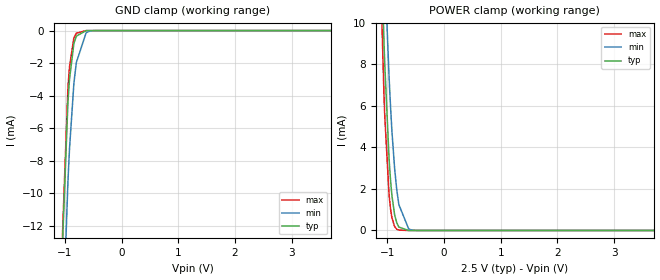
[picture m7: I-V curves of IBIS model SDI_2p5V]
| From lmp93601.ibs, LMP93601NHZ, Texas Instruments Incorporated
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|   Model SDI_2p5V
[Model]   SDI_2p5V
Model_type   Input
Vinl = 0.675
Vinh = 1.925
|   typ   min   max
|   (nom PVT)   (fast PVT)   (slow PVT)
C_comp   0.1436pF   0.1360pF   0.1525pF
[Model spec]
|subparameter
Vinl   0.75   0.675   0.825
Vinh   1.75   1.575   1.925
[Voltage Range]   2.5   2.25   2.75
[Temperature Range]   27   125   -25
[Power Clamp Reference]   2.5   2.25   2.75
[GND Clamp Reference]   0   0   0
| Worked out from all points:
|   GND clamp passes 1 mA (typ) near -0.85 V on its own axis
|   POWER clamp passes 1 mA (typ) near -0.88 V on its own axis
[GND Clamp]
|   Voltage   I(typ)   I(min)   I(max)
-2.5V     -336.2mA   -303.6mA   -362.1mA
-1.045V   -13.68mA   -19.4mA    -13.1mA
-1.038V   -12.76mA   -18.5mA    -12.11mA
-947.5mV  -4.564mA   -9.466mA   -3.67mA
-940mV    -4.119mA   -8.873mA   -3.25mA
-917.5mV  -2.979mA   -7.242mA   -2.208mA
-842.5mV  -847.5uA   -3.346mA   -480.3uA
-835mV    -735.5uA   -3.073mA   -404.1uA
-797.5mV  -344.8uA   -1.962mA   -161uA
-625mV    -3.072uA   -142.4uA   -461.6nA
-520mV    -77.11nA   -15.71uA   -2.842nA
4.992V    0A         0A         0A
[POWER Clamp]
|   Voltage   I(typ)   I(min)   I(max)
-2.5V     204.2mA    188.6mA    214.4mA
-1.157V   18.25mA    22.37mA    15.88mA
-1.06V    9.115mA    13.71mA    6.563mA
-1.045V   7.958mA    12.53mA    5.472mA
-970mV    3.467mA    7.411mA    1.731mA
-947.5mV  2.56mA     6.16mA     1.126mA
-872.5mV  767.8uA    3.005mA    193.9uA
-835mV    372.6uA    1.977mA    63.34uA
-797.5mV  163.8uA    1.248mA    17.13uA
-625mV    848.8nA    80.83uA    8.824nA
-542.5mV  40.15nA    13.45uA    0A
4.992V    0A         0A         0A
